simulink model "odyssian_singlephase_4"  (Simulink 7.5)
settings: Solver=ode23t  StartTime=0.0  StopTime=6  RelTol=1e-6
undefined symbols (not defined in the file or in its folder): dfilt, DiscIntNeverNeededParam
libraries: powerlib x72, powerlib_extras x29, simulink x24, dsparch4 x4
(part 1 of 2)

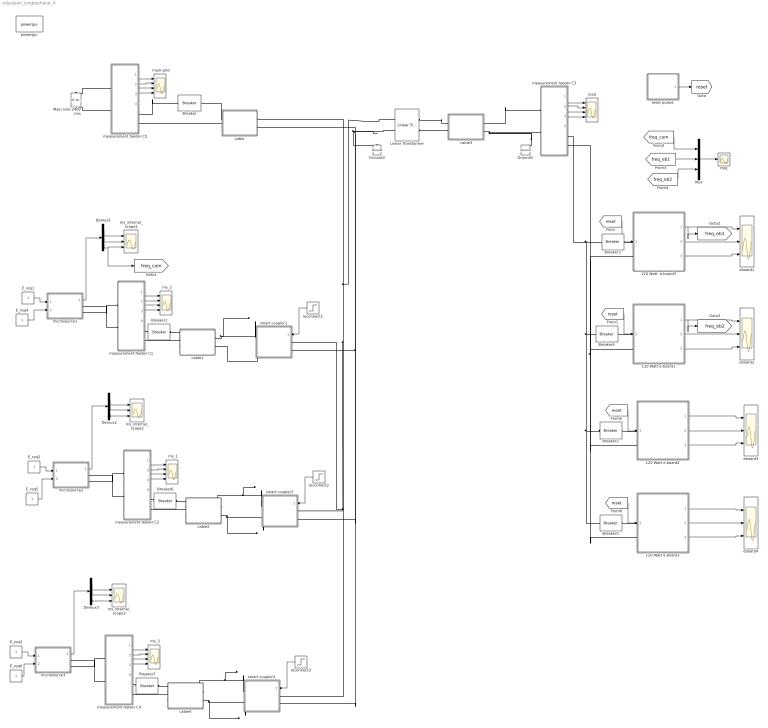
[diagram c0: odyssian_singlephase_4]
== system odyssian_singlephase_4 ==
  " load" : Scope  NumInputPorts=4
  " main-grid" : Scope  NumInputPorts=4
  " ms_1" : Scope  NumInputPorts=4
  " ms_2" : Scope  NumInputPorts=4
  " ms_3" : Scope  NumInputPorts=4
  120 Watt  e-board3 : Subsystem  mask{tf=100, p=1}
      mask prompts: tf "fault_time"; p "load priority"
  120 Watt e-board1 : Subsystem  mask{tf=100, p=1}
      mask prompts: tf "fault_time"; p "load priority"
  120 Watt e-board2 : Subsystem  mask{tf=100, p=1}
      mask prompts: tf "fault_time"; p "load priority"
  120 Watt e-board3 : Subsystem  mask{tf=100, p=2}
      mask prompts: tf "fault_time"; p "load priority"
  Breaker : powerlib/Elements/Breaker  DialogController=POWERSYS.PowerSysDialog  SystemSampleTime=-1  BreakerResistance=0.01  InitialState=1  SnubberResistance=1e6  SnubberCapacitance=inf  SwitchingTimes=[3]  External=off  Measurements=None  MoreParameters=off  NoBreakLoop=off
  Breaker{1..6} (6 alike) : powerlib/Elements/Breaker  DialogController=POWERSYS.PowerSysDialog  SystemSampleTime=-1  BreakerResistance=0.01  InitialState=1  SnubberResistance=1e6  SnubberCapacitance=inf  SwitchingTimes=[100]  External=off  Measurements=None  MoreParameters=off  NoBreakLoop=off
  Breaker7 : powerlib/Elements/Breaker  DialogController=POWERSYS.PowerSysDialog  SystemSampleTime=-1  BreakerResistance=0.01  InitialState=1  SnubberResistance=1e6  SnubberCapacitance=inf  SwitchingTimes=[4]  External=off  Measurements=None  MoreParameters=off  NoBreakLoop=off
  Demux1 : Demux  Outputs=3
  Demux2 : Demux  Outputs=3
  Demux3 : Demux  Outputs=3
  E_req{1..6} (6 alike) : Constant  OutDataType=fixdt(1, 16)  OutScaling=2^0
  Ground1 : powerlib/Elements/Ground  DialogController=POWERSYS.PowerSysDialog  PhysicalDomain=powersysdomain  SubClassName=unknown  LeftPortType=p1  RightPortType=p1  LConnTagsString=a
  Ground3 : powerlib/Elements/Ground  DialogController=POWERSYS.PowerSysDialog  PhysicalDomain=powersysdomain  SubClassName=unknown  LeftPortType=p1  RightPortType=p1  LConnTagsString=a
  Linear Transformer : powerlib/Elements/Linear Transformer  DialogController=POWERSYS.PowerSysDialog  PhysicalDomain=powersysdomain  SubClassName=unknown  LeftPortType=p1  RightPortType=p1  LConnTagsString=a|b  RConnTagsString=A|B  UNITS=SI  NominalPower=[ 45e3 , 60 ]  winding1=[240 0.001 1.e-3]  winding2=[120 .001 1.e-3]  ThreeWindings=off  winding3=[3.15e+05 0.7938 0.084225]  RmLm=[1.0804e+06 2866]  Measurements=All voltages and currents  DataType=on
  Main Grid 240V rms : powerlib/Electrical Sources/AC Voltage Source  DialogController=POWERSYS.PowerSysDialog  SystemSampleTime=-1  Amplitude=240*sqrt(2)  Phase=0  Frequency=60  SampleTime=0  Measurements=None
  Mux : Mux  Inputs=3
  cable : Subsystem
  cable1 : Subsystem
  cable2 : Subsystem
  cable3 : Subsystem
  cable4 : Subsystem
  eboard{1..4} (4 alike) : Scope  NumInputPorts=3
  freq : Scope
  measurement feeder C1 : Subsystem
  measurement feeder C2 : Subsystem
  measurement feeder C3 : Subsystem
  measurement feeder C4 : Subsystem
  measurement feeder C5 : Subsystem
  microsource1 : Subsystem  AncestorBlock=|
      | UWM_blocks/inverter-based
      | DG (simplified)
      | 208V - 15kVA
  microsource2 : Subsystem  AncestorBlock=|
      | UWM_blocks/inverter-based
      | DG (simplified)
      | 208V - 15kVA
  microsource3 : Subsystem  AncestorBlock=|
      | UWM_blocks/inverter-based
      | DG (simplified)
      | 208V - 15kVA
  ms_internal_scope1 : Scope  NumInputPorts=3
  ms_internal_scope2 : Scope  NumInputPorts=3
  ms_internal_scope3 : Scope  NumInputPorts=3
  powergui : powerlib/powergui  Priority=1  SystemSampleTime=-1  SimulationMode=Discrete  SampleTime=50e-5  frequency=60  SPID=off  DisableSnubberDevices=off  DisableRonSwitches=off  DisableVfSwitches=off  SwTol=0  Interpol=off  frequencyindice=0  echomessages=off  HookPort=off  DisplayEquations=off  FunctionMessages=off  EnableUseOfTLC=off  x0status=blocks  RestoreLinks=warning  ResistiveCurrentMeasurement=off  Frange=[0:2:500]  Ylog=off  Xlog=on  ShowGrid=off  save=off  variable=ZData  ZoomFFT=on  StartTime=0.0  cycles=1  DisplayStyle=1  fundamental=60  FreqAxis=off  MaxFrequency=1000  frequencyindicesteady=1  RmsSteady=1  display=off  Ts=0  methode=off
  reconnect1 : Step  Time=.1  SampleTime=0
  reconnect2 : Step  Time=.1  SampleTime=0
  reconnect3 : Step  Time=.1  SampleTime=0
  reset pulses : Subsystem  mask{tpulse=[50 100]}
  smart coupler1 : Subsystem
  smart coupler2 : Subsystem
  smart coupler3 : Subsystem
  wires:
  measurement feeder C3/1(Vm) -> " load"/1
  measurement feeder C3/2(Im) -> " load"/2
  measurement feeder C3/3(PQ) -> " load"/3
  measurement feeder C3/4(RMS (V-I)) -> " load"/4
  120 Watt  e-board3/1(w) -> eboard1/1, [freq_eb1]
  120 Watt  e-board3/2(Irms) -> eboard1/2
  120 Watt  e-board3/3(Vrms) -> eboard1/3
  [reset] -> 120 Watt  e-board3/1(reset)
  120 Watt e-board1/1(w) -> eboard2/1, [freq_eb2]
  120 Watt e-board1/2(Irms) -> eboard2/2
  120 Watt e-board1/3(Vrms) -> eboard2/3
  [reset] -> 120 Watt e-board1/1(reset)
  Mux/1 -> freq/1
  reset pulses/1(Out1) -> [reset]
  [freq_com] -> Mux/1
  [freq_eb1] -> Mux/2
  [freq_eb2] -> Mux/3
  measurement feeder C5/1(Vm) -> " main-grid"/1
  measurement feeder C5/2(Im) -> " main-grid"/2
  measurement feeder C5/3(PQ) -> " main-grid"/3
  measurement feeder C5/4(RMS (V-I)) -> " main-grid"/4
  measurement feeder C1/1(Vm) -> " ms_2"/1
  measurement feeder C1/2(Im) -> " ms_2"/2
  measurement feeder C1/3(PQ) -> " ms_2"/3
  measurement feeder C1/4(RMS (V-I)) -> " ms_2"/4
  E_req1/1 -> microsource1/1(E_req)
  Demux1/2 -> ms_internal_scope1/2
  Demux1/1 -> ms_internal_scope1/1
  Demux1/3 -> ms_internal_scope1/3, [freq_com]
  microsource1/1(m) -> Demux1/1
  reconnect1/1 -> smart coupler1/1(switch)
  ? -> ?
  120 Watt e-board2/1(w) -> eboard3/1
  120 Watt e-board2/2(Irms) -> eboard3/2
  120 Watt e-board2/3(Vrms) -> eboard3/3
  [reset] -> 120 Watt e-board2/1(reset)
  120 Watt e-board3/1(w) -> eboard4/1
  120 Watt e-board3/2(Irms) -> eboard4/2
  120 Watt e-board3/3(Vrms) -> eboard4/3
  [reset] -> 120 Watt e-board3/1(reset)
  measurement feeder C2/1(Vm) -> " ms_1"/1
  measurement feeder C2/2(Im) -> " ms_1"/2
  measurement feeder C2/3(PQ) -> " ms_1"/3
  measurement feeder C2/4(RMS (V-I)) -> " ms_1"/4
  E_req2/1 -> microsource2/1(E_req)
  Demux2/2 -> ms_internal_scope2/2
  Demux2/1 -> ms_internal_scope2/1
  Demux2/3 -> ms_internal_scope2/3
  microsource2/1(m) -> Demux2/1
  reconnect2/1 -> smart coupler2/1(switch)
  measurement feeder C4/1(Vm) -> " ms_3"/1
  measurement feeder C4/2(Im) -> " ms_3"/2
  measurement feeder C4/3(PQ) -> " ms_3"/3
  measurement feeder C4/4(RMS (V-I)) -> " ms_3"/4
  E_req3/1 -> microsource3/1(E_req)
  Demux3/2 -> ms_internal_scope3/2
  Demux3/1 -> ms_internal_scope3/1
  Demux3/3 -> ms_internal_scope3/3
  microsource3/1(m) -> Demux3/1
  reconnect3/1 -> smart coupler3/1(switch)
  E_req4/1 -> microsource1/2(P_req)
  E_req5/1 -> microsource2/2(P_req)
  E_req6/1 -> microsource3/2(P_req)
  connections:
  Breaker2/RConn1 -- Breaker4/RConn1 -- measurement feeder C3/RConn1 -- Breaker3/RConn1 -- Breaker5/RConn1
  measurement feeder C3/RConn2 -- 120 Watt  e-board3/LConn2 -- 120 Watt e-board1/LConn2 -- 120 Watt e-board2/LConn2 -- 120 Watt e-board3/LConn2
  cable3/LConn2 -- Ground1/LConn1 -- measurement feeder C3/LConn2
  120 Watt  e-board3/LConn1 -- Breaker3/LConn1
  120 Watt e-board1/LConn1 -- Breaker4/LConn1
  measurement feeder C5/RConn1 -- Breaker/LConn1
  cable/RConn2 -- measurement feeder C5/RConn2
  cable/RConn1 -- Breaker/RConn1
  smart coupler1/LConn1 -- Linear Transformer/LConn1 -- cable/LConn1 -- smart coupler2/LConn1 -- smart coupler3/LConn1
  Linear Transformer/LConn2 -- Ground3/LConn1 -- cable/LConn2 -- smart coupler1/LConn2 -- smart coupler2/LConn2 -- smart coupler3/LConn2
  cable3/LConn1 -- measurement feeder C3/LConn1
  cable3/RConn2 -- Linear Transformer/RConn2
  cable3/RConn1 -- Linear Transformer/RConn1
  measurement feeder C5/LConn1 -- Main Grid 240V rms/RConn1
  measurement feeder C5/LConn2 -- Main Grid 240V rms/LConn1
  smart coupler1/RConn2 -- cable1/LConn2
  cable1/LConn1 -- smart coupler1/RConn1
  cable1/RConn2 -- measurement feeder C1/RConn2
  measurement feeder C1/LConn1 -- microsource1/RConn1
  cable1/RConn1 -- Breaker1/LConn1
  measurement feeder C1/LConn2 -- microsource1/RConn2
  Breaker1/RConn1 -- measurement feeder C1/RConn1
  120 Watt e-board2/LConn1 -- Breaker2/LConn1
  120 Watt e-board3/LConn1 -- Breaker5/LConn1
  cable2/LConn2 -- smart coupler2/RConn2
  cable2/LConn1 -- smart coupler2/RConn1
  cable2/RConn2 -- measurement feeder C2/RConn2
  measurement feeder C2/LConn1 -- microsource2/RConn1
  cable2/RConn1 -- Breaker6/LConn1
  measurement feeder C2/LConn2 -- microsource2/RConn2
  Breaker6/RConn1 -- measurement feeder C2/RConn1
  cable4/LConn2 -- smart coupler3/RConn2
  cable4/LConn1 -- smart coupler3/RConn1
  cable4/RConn2 -- measurement feeder C4/RConn2
  measurement feeder C4/LConn1 -- microsource3/RConn1
  cable4/RConn1 -- Breaker7/LConn1
  measurement feeder C4/LConn2 -- microsource3/RConn2
  Breaker7/RConn1 -- measurement feeder C4/RConn1

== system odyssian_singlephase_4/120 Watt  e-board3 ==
  reset : Inport
  Breaker : powerlib/Elements/Breaker  DialogController=POWERSYS.PowerSysDialog  SystemSampleTime=-1  BreakerResistance=0.01  InitialState=1  SnubberResistance=1e6  SnubberCapacitance=inf  SwitchingTimes="[ 1/60  5/60 ]"  External=on  Measurements=None  MoreParameters=off  NoBreakLoop=off
  Current Measurement : powerlib/Measurements/Current Measurement  DialogController=POWERSYS.PowerSysDialog  SystemSampleTime=-1  PhasorSimulation=off  OutputType=Complex  PSBequivalent=0
  Ground : powerlib/Elements/Ground  DialogController=POWERSYS.PowerSysDialog  PhysicalDomain=powersysdomain  SubClassName=unknown  LeftPortType=p1  RightPortType=p1  LConnTagsString=a
  Series RLC Load : powerlib/Elements/Series RLC Load  DialogController=POWERSYS.PowerSysDialog  PhysicalDomain=powersysdomain  SubClassName=unknown  LeftPortType=p1  RightPortType=p1  LConnTagsString=a  RConnTagsString=__new0  NominalVoltage=120  NominalFrequency=60  ActivePower=120  InductivePower=0  CapacitivePower=0  Setx0=off  InitialVoltage=0  SetiL0=off  InitialCurrent=0  Measurements=None
  Voltage  Measurement : powerlib/Measurements/Voltage Measurement  DialogController=POWERSYS.PowerSysDialog  SystemSampleTime=-1  PhasorSimulation=off  OutputType=Complex  PSBequivalent=0
  trip : Subsystem  mask{p=p}
      mask prompts: p "priority level"
  A : PMIOPort  Port=1  Side=Left
  C : PMIOPort  Port=2  Side=Left
  w : Outport  OutDataType=fixdt(1, 16)  OutScaling=2^0
  Irms : Outport  Port=2  OutDataType=fixdt(1, 16)  OutScaling=2^0
  Vrms : Outport  Port=3  OutDataType=fixdt(1, 16)  OutScaling=2^0
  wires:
  trip/1(w) -> w/1
  Current Measurement/1 -> trip/3(I)
  Voltage  Measurement/1 -> trip/2(V)
  reset/1 -> trip/1(Reset)
  trip/2(trip) -> Breaker/1
  trip/3(Irms) -> Irms/1
  trip/4(Vrms) -> Vrms/1
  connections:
  A/RConn1 -- Current Measurement/LConn1 -- Voltage  Measurement/LConn1
  Voltage  Measurement/LConn2 -- Ground/LConn1
  Current Measurement/RConn1 -- Breaker/LConn1
  Series RLC Load/LConn1 -- Breaker/RConn1
  Series RLC Load/RConn1 -- C/RConn1

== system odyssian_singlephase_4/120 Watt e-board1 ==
  reset : Inport
  Breaker : powerlib/Elements/Breaker  DialogController=POWERSYS.PowerSysDialog  SystemSampleTime=-1  BreakerResistance=0.01  InitialState=1  SnubberResistance=1e6  SnubberCapacitance=inf  SwitchingTimes="[ 1/60  5/60 ]"  External=on  Measurements=None  MoreParameters=off  NoBreakLoop=off
  Current Measurement : powerlib/Measurements/Current Measurement  DialogController=POWERSYS.PowerSysDialog  SystemSampleTime=-1  PhasorSimulation=off  OutputType=Complex  PSBequivalent=0
  Ground : powerlib/Elements/Ground  DialogController=POWERSYS.PowerSysDialog  PhysicalDomain=powersysdomain  SubClassName=unknown  LeftPortType=p1  RightPortType=p1  LConnTagsString=a
  Series RLC Load : powerlib/Elements/Series RLC Load  DialogController=POWERSYS.PowerSysDialog  PhysicalDomain=powersysdomain  SubClassName=unknown  LeftPortType=p1  RightPortType=p1  LConnTagsString=a  RConnTagsString=__new0  NominalVoltage=120  NominalFrequency=60  ActivePower=120  InductivePower=0  CapacitivePower=0  Setx0=off  InitialVoltage=0  SetiL0=off  InitialCurrent=0  Measurements=None
  Voltage  Measurement : powerlib/Measurements/Voltage Measurement  DialogController=POWERSYS.PowerSysDialog  SystemSampleTime=-1  PhasorSimulation=off  OutputType=Complex  PSBequivalent=0
  trip : Subsystem  mask{p=p}
      mask prompts: p "priority level"
  A : PMIOPort  Port=1  Side=Left
  C : PMIOPort  Port=2  Side=Left
  w : Outport  OutDataType=fixdt(1, 16)  OutScaling=2^0
  Irms : Outport  Port=2  OutDataType=fixdt(1, 16)  OutScaling=2^0
  Vrms : Outport  Port=3  OutDataType=fixdt(1, 16)  OutScaling=2^0
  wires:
  trip/1(w) -> w/1
  Current Measurement/1 -> trip/3(I)
  Voltage  Measurement/1 -> trip/2(V)
  reset/1 -> trip/1(Reset)
  trip/2(trip) -> Breaker/1
  trip/3(Irms) -> Irms/1
  trip/4(Vrms) -> Vrms/1
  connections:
  A/RConn1 -- Current Measurement/LConn1 -- Voltage  Measurement/LConn1
  Voltage  Measurement/LConn2 -- Ground/LConn1
  Current Measurement/RConn1 -- Breaker/LConn1
  Series RLC Load/LConn1 -- Breaker/RConn1
  Series RLC Load/RConn1 -- C/RConn1

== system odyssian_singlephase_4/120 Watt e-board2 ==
  reset : Inport
  Breaker : powerlib/Elements/Breaker  DialogController=POWERSYS.PowerSysDialog  SystemSampleTime=-1  BreakerResistance=0.01  InitialState=1  SnubberResistance=1e6  SnubberCapacitance=inf  SwitchingTimes="[ 1/60  5/60 ]"  External=on  Measurements=None  MoreParameters=off  NoBreakLoop=off
  Current Measurement : powerlib/Measurements/Current Measurement  DialogController=POWERSYS.PowerSysDialog  SystemSampleTime=-1  PhasorSimulation=off  OutputType=Complex  PSBequivalent=0
  Ground : powerlib/Elements/Ground  DialogController=POWERSYS.PowerSysDialog  PhysicalDomain=powersysdomain  SubClassName=unknown  LeftPortType=p1  RightPortType=p1  LConnTagsString=a
  Series RLC Load : powerlib/Elements/Series RLC Load  DialogController=POWERSYS.PowerSysDialog  PhysicalDomain=powersysdomain  SubClassName=unknown  LeftPortType=p1  RightPortType=p1  LConnTagsString=a  RConnTagsString=__new0  NominalVoltage=120  NominalFrequency=60  ActivePower=120  InductivePower=0  CapacitivePower=0  Setx0=off  InitialVoltage=0  SetiL0=off  InitialCurrent=0  Measurements=None
  Voltage  Measurement : powerlib/Measurements/Voltage Measurement  DialogController=POWERSYS.PowerSysDialog  SystemSampleTime=-1  PhasorSimulation=off  OutputType=Complex  PSBequivalent=0
  trip : Subsystem  mask{p=p}
      mask prompts: p "priority level"
  A : PMIOPort  Port=1  Side=Left
  C : PMIOPort  Port=2  Side=Left
  w : Outport  OutDataType=fixdt(1, 16)  OutScaling=2^0
  Irms : Outport  Port=2  OutDataType=fixdt(1, 16)  OutScaling=2^0
  Vrms : Outport  Port=3  OutDataType=fixdt(1, 16)  OutScaling=2^0
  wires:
  trip/1(w) -> w/1
  Current Measurement/1 -> trip/3(I)
  Voltage  Measurement/1 -> trip/2(V)
  reset/1 -> trip/1(Reset)
  trip/2(trip) -> Breaker/1
  trip/3(Irms) -> Irms/1
  trip/4(Vrms) -> Vrms/1
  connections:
  A/RConn1 -- Current Measurement/LConn1 -- Voltage  Measurement/LConn1
  Voltage  Measurement/LConn2 -- Ground/LConn1
  Current Measurement/RConn1 -- Breaker/LConn1
  Series RLC Load/LConn1 -- Breaker/RConn1
  Series RLC Load/RConn1 -- C/RConn1

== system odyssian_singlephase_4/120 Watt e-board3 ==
  reset : Inport
  Breaker : powerlib/Elements/Breaker  DialogController=POWERSYS.PowerSysDialog  SystemSampleTime=-1  BreakerResistance=0.01  InitialState=1  SnubberResistance=1e6  SnubberCapacitance=inf  SwitchingTimes="[ 1/60  5/60 ]"  External=on  Measurements=None  MoreParameters=off  NoBreakLoop=off
  Current Measurement : powerlib/Measurements/Current Measurement  DialogController=POWERSYS.PowerSysDialog  SystemSampleTime=-1  PhasorSimulation=off  OutputType=Complex  PSBequivalent=0
  Ground : powerlib/Elements/Ground  DialogController=POWERSYS.PowerSysDialog  PhysicalDomain=powersysdomain  SubClassName=unknown  LeftPortType=p1  RightPortType=p1  LConnTagsString=a
  Series RLC Load : powerlib/Elements/Series RLC Load  DialogController=POWERSYS.PowerSysDialog  PhysicalDomain=powersysdomain  SubClassName=unknown  LeftPortType=p1  RightPortType=p1  LConnTagsString=a  RConnTagsString=__new0  NominalVoltage=120  NominalFrequency=60  ActivePower=120  InductivePower=0  CapacitivePower=0  Setx0=off  InitialVoltage=0  SetiL0=off  InitialCurrent=0  Measurements=None
  Voltage  Measurement : powerlib/Measurements/Voltage Measurement  DialogController=POWERSYS.PowerSysDialog  SystemSampleTime=-1  PhasorSimulation=off  OutputType=Complex  PSBequivalent=0
  trip : Subsystem  mask{p=p}
      mask prompts: p "priority level"
  A : PMIOPort  Port=1  Side=Left
  C : PMIOPort  Port=2  Side=Left
  w : Outport  OutDataType=fixdt(1, 16)  OutScaling=2^0
  Irms : Outport  Port=2  OutDataType=fixdt(1, 16)  OutScaling=2^0
  Vrms : Outport  Port=3  OutDataType=fixdt(1, 16)  OutScaling=2^0
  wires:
  trip/1(w) -> w/1
  Current Measurement/1 -> trip/3(I)
  Voltage  Measurement/1 -> trip/2(V)
  reset/1 -> trip/1(Reset)
  trip/2(trip) -> Breaker/1
  trip/3(Irms) -> Irms/1
  trip/4(Vrms) -> Vrms/1
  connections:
  A/RConn1 -- Current Measurement/LConn1 -- Voltage  Measurement/LConn1
  Voltage  Measurement/LConn2 -- Ground/LConn1
  Current Measurement/RConn1 -- Breaker/LConn1
  Series RLC Load/LConn1 -- Breaker/RConn1
  Series RLC Load/RConn1 -- C/RConn1

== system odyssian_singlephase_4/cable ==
  Series RLC Branch : powerlib/Elements/Series RLC Branch  DialogController=POWERSYS.PowerSysDialog  PhysicalDomain=powersysdomain  SubClassName=unknown  LeftPortType=p1  RightPortType=p1  LConnTagsString=__new0  RConnTagsString=__new0  BranchType=RL  Resistance=.001  Inductance=1.e-5  SetiL0=off  InitialCurrent=0  Capacitance=1e-6  Setx0=off  InitialVoltage=0  Measurements=None
  A : PMIOPort  Tag=PMCPort  Port=1  Side=Left
  A' : PMIOPort  Tag=PMCPort  Port=2  Side=Right
  B' : PMIOPort  Tag=PMCPort  Port=3  Side=Right
  B : PMIOPort  Tag=PMCPort  Port=4  Side=Left
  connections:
  A/RConn1 -- Series RLC Branch/LConn1
  A'/RConn1 -- Series RLC Branch/RConn1
  B/RConn1 -- B'/RConn1

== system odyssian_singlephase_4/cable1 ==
  Series RLC Branch : powerlib/Elements/Series RLC Branch  DialogController=POWERSYS.PowerSysDialog  PhysicalDomain=powersysdomain  SubClassName=unknown  LeftPortType=p1  RightPortType=p1  LConnTagsString=__new0  RConnTagsString=__new0  BranchType=RL  Resistance=.001  Inductance=1.e-6  SetiL0=off  InitialCurrent=0  Capacitance=1e-6  Setx0=off  InitialVoltage=0  Measurements=None
  A : PMIOPort  Tag=PMCPort  Port=1  Side=Left
  A' : PMIOPort  Tag=PMCPort  Port=2  Side=Right
  B' : PMIOPort  Tag=PMCPort  Port=3  Side=Right
  B : PMIOPort  Tag=PMCPort  Port=4  Side=Left
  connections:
  A/RConn1 -- Series RLC Branch/LConn1
  Series RLC Branch/RConn1 -- A'/RConn1
  B/RConn1 -- B'/RConn1

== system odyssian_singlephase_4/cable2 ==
  Series RLC Branch : powerlib/Elements/Series RLC Branch  DialogController=POWERSYS.PowerSysDialog  PhysicalDomain=powersysdomain  SubClassName=unknown  LeftPortType=p1  RightPortType=p1  LConnTagsString=__new0  RConnTagsString=__new0  BranchType=RL  Resistance=.001  Inductance=1.e-6  SetiL0=off  InitialCurrent=0  Capacitance=1e-6  Setx0=off  InitialVoltage=0  Measurements=None
  A : PMIOPort  Tag=PMCPort  Port=1  Side=Left
  A' : PMIOPort  Tag=PMCPort  Port=2  Side=Right
  B' : PMIOPort  Tag=PMCPort  Port=3  Side=Right
  B : PMIOPort  Tag=PMCPort  Port=4  Side=Left
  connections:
  A/RConn1 -- Series RLC Branch/LConn1
  Series RLC Branch/RConn1 -- A'/RConn1
  B/RConn1 -- B'/RConn1

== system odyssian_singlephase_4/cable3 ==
  Series RLC Branch : powerlib/Elements/Series RLC Branch  DialogController=POWERSYS.PowerSysDialog  PhysicalDomain=powersysdomain  SubClassName=unknown  LeftPortType=p1  RightPortType=p1  LConnTagsString=__new0  RConnTagsString=__new0  BranchType=RL  Resistance=.001  Inductance=1.e-6  SetiL0=off  InitialCurrent=0  Capacitance=1e-6  Setx0=off  InitialVoltage=0  Measurements=None
  A : PMIOPort  Tag=PMCPort  Port=1  Side=Left
  A' : PMIOPort  Tag=PMCPort  Port=2  Side=Right
  B' : PMIOPort  Tag=PMCPort  Port=3  Side=Right
  B : PMIOPort  Tag=PMCPort  Port=4  Side=Left
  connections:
  A/RConn1 -- Series RLC Branch/LConn1
  Series RLC Branch/RConn1 -- A'/RConn1
  B/RConn1 -- B'/RConn1

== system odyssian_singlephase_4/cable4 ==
  Series RLC Branch : powerlib/Elements/Series RLC Branch  DialogController=POWERSYS.PowerSysDialog  PhysicalDomain=powersysdomain  SubClassName=unknown  LeftPortType=p1  RightPortType=p1  LConnTagsString=__new0  RConnTagsString=__new0  BranchType=RL  Resistance=.001  Inductance=1.e-6  SetiL0=off  InitialCurrent=0  Capacitance=1e-6  Setx0=off  InitialVoltage=0  Measurements=None
  A : PMIOPort  Tag=PMCPort  Port=1  Side=Left
  A' : PMIOPort  Tag=PMCPort  Port=2  Side=Right
  B' : PMIOPort  Tag=PMCPort  Port=3  Side=Right
  B : PMIOPort  Tag=PMCPort  Port=4  Side=Left
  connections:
  A/RConn1 -- Series RLC Branch/LConn1
  Series RLC Branch/RConn1 -- A'/RConn1
  B/RConn1 -- B'/RConn1

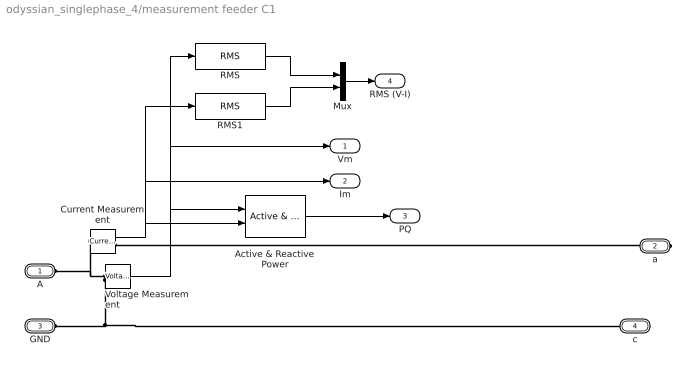
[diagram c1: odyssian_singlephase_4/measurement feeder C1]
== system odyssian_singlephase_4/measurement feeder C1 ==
  Active & Reactive Power : powerlib_extras/Measurements/Active & Reactive Power  DialogController=POWERSYS.PowerSysDialog  SystemSampleTime=-1  f1=60
  Current Measurement : powerlib/Measurements/Current Measurement  DialogController=POWERSYS.PowerSysDialog  SystemSampleTime=-1  PhasorSimulation=off  OutputType=Complex  PSBequivalent=0
  Mux : Mux  Inputs=2
  RMS : powerlib_extras/Measurements/RMS  DialogController=POWERSYS.PowerSysDialog  SystemSampleTime=-1  f1=60
  RMS1 : powerlib_extras/Measurements/RMS  DialogController=POWERSYS.PowerSysDialog  SystemSampleTime=-1  f1=60
  Voltage Measurement : powerlib/Measurements/Voltage Measurement  DialogController=POWERSYS.PowerSysDialog  SystemSampleTime=-1  PhasorSimulation=off  OutputType=Complex  PSBequivalent=0
  A : PMIOPort  Port=1  Side=Left
  a : PMIOPort  Port=2  Side=Right
  GND : PMIOPort  Port=3  Side=Left
  c : PMIOPort  Port=4  Side=Right
  Vm : Outport  OutDataType=fixdt(1, 16)  OutScaling=2^0
  Im : Outport  Port=2  OutDataType=fixdt(1, 16)  OutScaling=2^0
  PQ : Outport  Port=3  OutDataType=fixdt(1, 16)  OutScaling=2^0
  RMS (V-I) : Outport  Port=4  OutDataType=fixdt(1, 16)  OutScaling=2^0
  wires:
  Mux/1 -> RMS (V-I)/1
  Current Measurement/1 -> Im/1, RMS1/1, Active & Reactive Power/2
  Voltage Measurement/1 -> Vm/1, RMS/1, Active & Reactive Power/1
  Active & Reactive Power/1 -> PQ/1
  RMS/1 -> Mux/1
  RMS1/1 -> Mux/2
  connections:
  a/RConn1 -- Current Measurement/RConn1
  Voltage Measurement/LConn1 -- A/RConn1 -- Current Measurement/LConn1
  Voltage Measurement/LConn2 -- GND/RConn1 -- c/RConn1

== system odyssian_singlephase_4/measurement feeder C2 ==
  Active & Reactive Power : powerlib_extras/Measurements/Active & Reactive Power  DialogController=POWERSYS.PowerSysDialog  SystemSampleTime=-1  f1=60
  Current Measurement : powerlib/Measurements/Current Measurement  DialogController=POWERSYS.PowerSysDialog  SystemSampleTime=-1  PhasorSimulation=off  OutputType=Complex  PSBequivalent=0
  Mux : Mux  Inputs=2
  RMS : powerlib_extras/Measurements/RMS  DialogController=POWERSYS.PowerSysDialog  SystemSampleTime=-1  f1=60
  RMS1 : powerlib_extras/Measurements/RMS  DialogController=POWERSYS.PowerSysDialog  SystemSampleTime=-1  f1=60
  Voltage Measurement : powerlib/Measurements/Voltage Measurement  DialogController=POWERSYS.PowerSysDialog  SystemSampleTime=-1  PhasorSimulation=off  OutputType=Complex  PSBequivalent=0
  A : PMIOPort  Port=1  Side=Left
  a : PMIOPort  Port=2  Side=Right
  GND : PMIOPort  Port=3  Side=Left
  c : PMIOPort  Port=4  Side=Right
  Vm : Outport  OutDataType=fixdt(1, 16)  OutScaling=2^0
  Im : Outport  Port=2  OutDataType=fixdt(1, 16)  OutScaling=2^0
  PQ : Outport  Port=3  OutDataType=fixdt(1, 16)  OutScaling=2^0
  RMS (V-I) : Outport  Port=4  OutDataType=fixdt(1, 16)  OutScaling=2^0
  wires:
  Mux/1 -> RMS (V-I)/1
  Current Measurement/1 -> Im/1, RMS1/1, Active & Reactive Power/2
  Voltage Measurement/1 -> Vm/1, RMS/1, Active & Reactive Power/1
  Active & Reactive Power/1 -> PQ/1
  RMS/1 -> Mux/1
  RMS1/1 -> Mux/2
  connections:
  a/RConn1 -- Current Measurement/RConn1
  Voltage Measurement/LConn1 -- A/RConn1 -- Current Measurement/LConn1
  Voltage Measurement/LConn2 -- GND/RConn1 -- c/RConn1

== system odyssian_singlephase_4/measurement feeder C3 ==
  Active & Reactive Power : powerlib_extras/Measurements/Active & Reactive Power  DialogController=POWERSYS.PowerSysDialog  SystemSampleTime=-1  f1=60
  Current Measurement : powerlib/Measurements/Current Measurement  DialogController=POWERSYS.PowerSysDialog  SystemSampleTime=-1  PhasorSimulation=off  OutputType=Complex  PSBequivalent=0
  Mux : Mux  Inputs=2
  RMS : powerlib_extras/Measurements/RMS  DialogController=POWERSYS.PowerSysDialog  SystemSampleTime=-1  f1=60
  RMS1 : powerlib_extras/Measurements/RMS  DialogController=POWERSYS.PowerSysDialog  SystemSampleTime=-1  f1=60
  Voltage Measurement : powerlib/Measurements/Voltage Measurement  DialogController=POWERSYS.PowerSysDialog  SystemSampleTime=-1  PhasorSimulation=off  OutputType=Complex  PSBequivalent=0
  A : PMIOPort  Port=1  Side=Left
  a : PMIOPort  Port=2  Side=Right
  GND : PMIOPort  Port=3  Side=Left
  c : PMIOPort  Port=4  Side=Right
  Vm : Outport  OutDataType=fixdt(1, 16)  OutScaling=2^0
  Im : Outport  Port=2  OutDataType=fixdt(1, 16)  OutScaling=2^0
  PQ : Outport  Port=3  OutDataType=fixdt(1, 16)  OutScaling=2^0
  RMS (V-I) : Outport  Port=4  OutDataType=fixdt(1, 16)  OutScaling=2^0
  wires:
  Mux/1 -> RMS (V-I)/1
  Current Measurement/1 -> Im/1, RMS1/1, Active & Reactive Power/2
  Voltage Measurement/1 -> Vm/1, RMS/1, Active & Reactive Power/1
  Active & Reactive Power/1 -> PQ/1
  RMS/1 -> Mux/1
  RMS1/1 -> Mux/2
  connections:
  a/RConn1 -- Current Measurement/RConn1
  Voltage Measurement/LConn1 -- A/RConn1 -- Current Measurement/LConn1
  Voltage Measurement/LConn2 -- GND/RConn1 -- c/RConn1

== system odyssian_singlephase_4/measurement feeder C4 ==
  Active & Reactive Power : powerlib_extras/Measurements/Active & Reactive Power  DialogController=POWERSYS.PowerSysDialog  SystemSampleTime=-1  f1=60
  Current Measurement : powerlib/Measurements/Current Measurement  DialogController=POWERSYS.PowerSysDialog  SystemSampleTime=-1  PhasorSimulation=off  OutputType=Complex  PSBequivalent=0
  Mux : Mux  Inputs=2
  RMS : powerlib_extras/Measurements/RMS  DialogController=POWERSYS.PowerSysDialog  SystemSampleTime=-1  f1=60
  RMS1 : powerlib_extras/Measurements/RMS  DialogController=POWERSYS.PowerSysDialog  SystemSampleTime=-1  f1=60
  Voltage Measurement : powerlib/Measurements/Voltage Measurement  DialogController=POWERSYS.PowerSysDialog  SystemSampleTime=-1  PhasorSimulation=off  OutputType=Complex  PSBequivalent=0
  A : PMIOPort  Port=1  Side=Left
  a : PMIOPort  Port=2  Side=Right
  GND : PMIOPort  Port=3  Side=Left
  c : PMIOPort  Port=4  Side=Right
  Vm : Outport  OutDataType=fixdt(1, 16)  OutScaling=2^0
  Im : Outport  Port=2  OutDataType=fixdt(1, 16)  OutScaling=2^0
  PQ : Outport  Port=3  OutDataType=fixdt(1, 16)  OutScaling=2^0
  RMS (V-I) : Outport  Port=4  OutDataType=fixdt(1, 16)  OutScaling=2^0
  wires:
  Mux/1 -> RMS (V-I)/1
  Current Measurement/1 -> Im/1, RMS1/1, Active & Reactive Power/2
  Voltage Measurement/1 -> Vm/1, RMS/1, Active & Reactive Power/1
  Active & Reactive Power/1 -> PQ/1
  RMS/1 -> Mux/1
  RMS1/1 -> Mux/2
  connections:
  a/RConn1 -- Current Measurement/RConn1
  Voltage Measurement/LConn1 -- A/RConn1 -- Current Measurement/LConn1
  Voltage Measurement/LConn2 -- GND/RConn1 -- c/RConn1

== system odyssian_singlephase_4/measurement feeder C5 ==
  Active & Reactive Power : powerlib_extras/Measurements/Active & Reactive Power  DialogController=POWERSYS.PowerSysDialog  SystemSampleTime=-1  f1=60
  Current Measurement : powerlib/Measurements/Current Measurement  DialogController=POWERSYS.PowerSysDialog  SystemSampleTime=-1  PhasorSimulation=off  OutputType=Complex  PSBequivalent=0
  Mux : Mux  Inputs=2
  RMS : powerlib_extras/Measurements/RMS  DialogController=POWERSYS.PowerSysDialog  SystemSampleTime=-1  f1=60
  RMS1 : powerlib_extras/Measurements/RMS  DialogController=POWERSYS.PowerSysDialog  SystemSampleTime=-1  f1=60
  Voltage Measurement : powerlib/Measurements/Voltage Measurement  DialogController=POWERSYS.PowerSysDialog  SystemSampleTime=-1  PhasorSimulation=off  OutputType=Complex  PSBequivalent=0
  A : PMIOPort  Port=1  Side=Left
  a : PMIOPort  Port=2  Side=Right
  GND : PMIOPort  Port=3  Side=Left
  c : PMIOPort  Port=4  Side=Right
  Vm : Outport  OutDataType=fixdt(1, 16)  OutScaling=2^0
  Im : Outport  Port=2  OutDataType=fixdt(1, 16)  OutScaling=2^0
  PQ : Outport  Port=3  OutDataType=fixdt(1, 16)  OutScaling=2^0
  RMS (V-I) : Outport  Port=4  OutDataType=fixdt(1, 16)  OutScaling=2^0
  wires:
  Mux/1 -> RMS (V-I)/1
  Current Measurement/1 -> Im/1, RMS1/1, Active & Reactive Power/2
  Voltage Measurement/1 -> Vm/1, RMS/1, Active & Reactive Power/1
  Active & Reactive Power/1 -> PQ/1
  RMS/1 -> Mux/1
  RMS1/1 -> Mux/2
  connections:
  a/RConn1 -- Current Measurement/RConn1
  Voltage Measurement/LConn1 -- A/RConn1 -- Current Measurement/LConn1
  Voltage Measurement/LConn2 -- GND/RConn1 -- c/RConn1

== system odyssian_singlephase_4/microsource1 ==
  E_req : Inport
  P_req : Inport  Port=2
  Current Measurement : powerlib/Measurements/Current Measurement  DialogController=POWERSYS.PowerSysDialog  SystemSampleTime=-1  PhasorSimulation=off  OutputType=Complex  PSBequivalent=0
  Gain : Gain  Gain=1/(2*pi)  ParameterDataType=fixdt(1, 16)  ParameterScaling=2^0  OutDataType=fixdt(1, 16)  OutScaling=2^0
  Mux : Mux  Inputs=3
  Parallel RLC Branch : powerlib/Elements/Parallel RLC Branch  DialogController=POWERSYS.PowerSysDialog  PhysicalDomain=powersysdomain  SubClassName=unknown  LeftPortType=p1  RightPortType=p1  LConnTagsString=a  RConnTagsString=__new0  BranchType=L  Resistance=1  Inductance=1.e-1  SetiL0=off  InitialCurrent=0  Capacitance=1e-6  Setx0=off  InitialVoltage=0  Measurements=None
  Parallel RLC Branch1 : powerlib/Elements/Parallel RLC Branch  DialogController=POWERSYS.PowerSysDialog  PhysicalDomain=powersysdomain  SubClassName=unknown  LeftPortType=p1  RightPortType=p1  LConnTagsString=a  RConnTagsString=__new0  BranchType=L  Resistance=1  Inductance=1.e-1  SetiL0=off  InitialCurrent=0  Capacitance=1e-6  Setx0=off  InitialVoltage=0  Measurements=None
  Parallel RLC Branch2 : powerlib/Elements/Parallel RLC Branch  DialogController=POWERSYS.PowerSysDialog  PhysicalDomain=powersysdomain  SubClassName=unknown  LeftPortType=p1  RightPortType=p1  LConnTagsString=a  RConnTagsString=__new0  BranchType=C  Resistance=1  Inductance=1.e-1  SetiL0=off  InitialCurrent=0  Capacitance=1.e-5  Setx0=off  InitialVoltage=0  Measurements=None
  UWM_controller : Subsystem  mask{Vbase=240*sqrt(2), Sbase=200}
  Voltage Measurement : powerlib/Measurements/Voltage Measurement  DialogController=POWERSYS.PowerSysDialog  SystemSampleTime=-1  PhasorSimulation=off  OutputType=Complex  PSBequivalent=0
  microsource : Subsystem
  a : PMIOPort  Port=1  Side=Right
  GND : PMIOPort  Port=2  Side=Right
  m : Outport  OutDataType=fixdt(1, 16)  OutScaling=2^0
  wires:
  E_req/1 -> UWM_controller/3(E_req)
  P_req/1 -> UWM_controller/4(P_req)
  UWM_controller/1(Vpk) -> microsource/1(Vpk)
  UWM_controller/2(w) -> microsource/2(w), Gain/1
  Mux/1 -> m/1
  Gain/1 -> Mux/3
  Current Measurement/1 -> Mux/2, UWM_controller/2(i_meas)
  Voltage Measurement/1 -> Mux/1, UWM_controller/1(v_meas)
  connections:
  Voltage Measurement/LConn2 -- GND/RConn1 -- Parallel RLC Branch2/RConn1 -- microsource/RConn2
  Parallel RLC Branch1/RConn1 -- Voltage Measurement/LConn1 -- Current Measurement/LConn1
  a/RConn1 -- Current Measurement/RConn1
  Parallel RLC Branch/LConn1 -- microsource/RConn1
  Parallel RLC Branch2/LConn1 -- Parallel RLC Branch1/LConn1 -- Parallel RLC Branch/RConn1

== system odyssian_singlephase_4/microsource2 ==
  E_req : Inport
  P_req : Inport  Port=2
  Current Measurement : powerlib/Measurements/Current Measurement  DialogController=POWERSYS.PowerSysDialog  SystemSampleTime=-1  PhasorSimulation=off  OutputType=Complex  PSBequivalent=0
  Gain : Gain  Gain=1/(2*pi)  ParameterDataType=fixdt(1, 16)  ParameterScaling=2^0  OutDataType=fixdt(1, 16)  OutScaling=2^0
  Mux : Mux  Inputs=3
  Parallel RLC Branch : powerlib/Elements/Parallel RLC Branch  DialogController=POWERSYS.PowerSysDialog  PhysicalDomain=powersysdomain  SubClassName=unknown  LeftPortType=p1  RightPortType=p1  LConnTagsString=a  RConnTagsString=__new0  BranchType=L  Resistance=1  Inductance=1.e-1  SetiL0=off  InitialCurrent=0  Capacitance=1e-6  Setx0=off  InitialVoltage=0  Measurements=None
  Parallel RLC Branch1 : powerlib/Elements/Parallel RLC Branch  DialogController=POWERSYS.PowerSysDialog  PhysicalDomain=powersysdomain  SubClassName=unknown  LeftPortType=p1  RightPortType=p1  LConnTagsString=a  RConnTagsString=__new0  BranchType=L  Resistance=1  Inductance=1.e-1  SetiL0=off  InitialCurrent=0  Capacitance=1e-6  Setx0=off  InitialVoltage=0  Measurements=None
  Parallel RLC Branch2 : powerlib/Elements/Parallel RLC Branch  DialogController=POWERSYS.PowerSysDialog  PhysicalDomain=powersysdomain  SubClassName=unknown  LeftPortType=p1  RightPortType=p1  LConnTagsString=a  RConnTagsString=__new0  BranchType=C  Resistance=1  Inductance=1.e-1  SetiL0=off  InitialCurrent=0  Capacitance=1.e-5  Setx0=off  InitialVoltage=0  Measurements=None
  UWM_controller : Subsystem  mask{Vbase=240*sqrt(2), Sbase=200}
  Voltage Measurement : powerlib/Measurements/Voltage Measurement  DialogController=POWERSYS.PowerSysDialog  SystemSampleTime=-1  PhasorSimulation=off  OutputType=Complex  PSBequivalent=0
  microsource : Subsystem
  a : PMIOPort  Port=1  Side=Right
  GND : PMIOPort  Port=2  Side=Right
  m : Outport  OutDataType=fixdt(1, 16)  OutScaling=2^0
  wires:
  E_req/1 -> UWM_controller/3(E_req)
  P_req/1 -> UWM_controller/4(P_req)
  UWM_controller/1(Vpk) -> microsource/1(Vpk)
  UWM_controller/2(w) -> microsource/2(w), Gain/1
  Mux/1 -> m/1
  Gain/1 -> Mux/3
  Current Measurement/1 -> Mux/2, UWM_controller/2(i_meas)
  Voltage Measurement/1 -> Mux/1, UWM_controller/1(v_meas)
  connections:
  Voltage Measurement/LConn2 -- GND/RConn1 -- Parallel RLC Branch2/RConn1 -- microsource/RConn2
  Parallel RLC Branch1/RConn1 -- Voltage Measurement/LConn1 -- Current Measurement/LConn1
  a/RConn1 -- Current Measurement/RConn1
  Parallel RLC Branch/LConn1 -- microsource/RConn1
  Parallel RLC Branch2/LConn1 -- Parallel RLC Branch1/LConn1 -- Parallel RLC Branch/RConn1

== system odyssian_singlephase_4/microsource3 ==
  E_req : Inport
  P_req : Inport  Port=2
  Current Measurement : powerlib/Measurements/Current Measurement  DialogController=POWERSYS.PowerSysDialog  SystemSampleTime=-1  PhasorSimulation=off  OutputType=Complex  PSBequivalent=0
  Gain : Gain  Gain=1/(2*pi)  ParameterDataType=fixdt(1, 16)  ParameterScaling=2^0  OutDataType=fixdt(1, 16)  OutScaling=2^0
  Mux : Mux  Inputs=3
  Parallel RLC Branch : powerlib/Elements/Parallel RLC Branch  DialogController=POWERSYS.PowerSysDialog  PhysicalDomain=powersysdomain  SubClassName=unknown  LeftPortType=p1  RightPortType=p1  LConnTagsString=a  RConnTagsString=__new0  BranchType=L  Resistance=1  Inductance=1.e-1  SetiL0=off  InitialCurrent=0  Capacitance=1e-6  Setx0=off  InitialVoltage=0  Measurements=None
  Parallel RLC Branch1 : powerlib/Elements/Parallel RLC Branch  DialogController=POWERSYS.PowerSysDialog  PhysicalDomain=powersysdomain  SubClassName=unknown  LeftPortType=p1  RightPortType=p1  LConnTagsString=a  RConnTagsString=__new0  BranchType=L  Resistance=1  Inductance=1.e-1  SetiL0=off  InitialCurrent=0  Capacitance=1e-6  Setx0=off  InitialVoltage=0  Measurements=None
  Parallel RLC Branch2 : powerlib/Elements/Parallel RLC Branch  DialogController=POWERSYS.PowerSysDialog  PhysicalDomain=powersysdomain  SubClassName=unknown  LeftPortType=p1  RightPortType=p1  LConnTagsString=a  RConnTagsString=__new0  BranchType=C  Resistance=1  Inductance=1.e-1  SetiL0=off  InitialCurrent=0  Capacitance=1.e-5  Setx0=off  InitialVoltage=0  Measurements=None
  UWM_controller : Subsystem  mask{Vbase=240*sqrt(2), Sbase=200}
  Voltage Measurement : powerlib/Measurements/Voltage Measurement  DialogController=POWERSYS.PowerSysDialog  SystemSampleTime=-1  PhasorSimulation=off  OutputType=Complex  PSBequivalent=0
  microsource : Subsystem
  a : PMIOPort  Port=1  Side=Right
  GND : PMIOPort  Port=2  Side=Right
  m : Outport  OutDataType=fixdt(1, 16)  OutScaling=2^0
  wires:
  E_req/1 -> UWM_controller/3(E_req)
  P_req/1 -> UWM_controller/4(P_req)
  UWM_controller/1(Vpk) -> microsource/1(Vpk)
  UWM_controller/2(w) -> microsource/2(w), Gain/1
  Mux/1 -> m/1
  Gain/1 -> Mux/3
  Current Measurement/1 -> Mux/2, UWM_controller/2(i_meas)
  Voltage Measurement/1 -> Mux/1, UWM_controller/1(v_meas)
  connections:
  Voltage Measurement/LConn2 -- GND/RConn1 -- Parallel RLC Branch2/RConn1 -- microsource/RConn2
  Parallel RLC Branch1/RConn1 -- Voltage Measurement/LConn1 -- Current Measurement/LConn1
  a/RConn1 -- Current Measurement/RConn1
  Parallel RLC Branch/LConn1 -- microsource/RConn1
  Parallel RLC Branch2/LConn1 -- Parallel RLC Branch1/LConn1 -- Parallel RLC Branch/RConn1

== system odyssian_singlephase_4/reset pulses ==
  Sum : Sum  Inputs=|++  OutDataType=fixdt(1, 16)  OutScaling=2^0
  pulse : Subsystem  mask{tstart=tpulse(1), dt=.1}
  pulse1 : Subsystem  mask{tstart=tpulse(2), dt=.1}
  Out1 : Outport
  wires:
  pulse/1(Out1) -> Sum/1
  pulse1/1(Out1) -> Sum/2
  Sum/1 -> Out1/1

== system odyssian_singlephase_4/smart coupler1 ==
  switch : Inport  OutDataType=fixdt(1, 16)  OutScaling=2^0
  Abs : Abs  OutDataType=fixdt(1, 16)  OutScaling=2^0
  Breaker : powerlib/Elements/Breaker  DialogController=POWERSYS.PowerSysDialog  SystemSampleTime=-1  BreakerResistance=0.01  InitialState=0  SnubberResistance=1e6  SnubberCapacitance=inf  SwitchingTimes="[ 1/60  5/60 ]"  External=on  Measurements=None  MoreParameters=off  NoBreakLoop=off
  Level-2 M-file S-Function : M-S-Function  FunctionName=smart_coupler
  Scope : Scope  NumInputPorts=3
  Transfer Fcn : TransferFcn  Numerator=[100]  Denominator=[1 100]
  Voltage Measurement : powerlib/Measurements/Voltage Measurement  DialogController=POWERSYS.PowerSysDialog  SystemSampleTime=-1  PhasorSimulation=off  OutputType=Complex  PSBequivalent=0
  A : PMIOPort  Port=1  Side=Left
  C : PMIOPort  Port=2  Side=Left
  a : PMIOPort  Port=3  Side=Right
  c : PMIOPort  Port=4  Side=Right
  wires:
  switch/1 -> Level-2 M-file S-Function/2, Scope/2
  Level-2 M-file S-Function/1 -> Scope/1, Breaker/1
  Voltage Measurement/1 -> Abs/1
  Abs/1 -> Transfer Fcn/1
  Transfer Fcn/1 -> Level-2 M-file S-Function/1, Scope/3
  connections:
  Breaker/LConn1 -- A/RConn1 -- Voltage Measurement/LConn1
  Breaker/RConn1 -- Voltage Measurement/LConn2 -- a/RConn1
  c/RConn1 -- C/RConn1

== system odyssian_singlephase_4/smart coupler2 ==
  switch : Inport  OutDataType=fixdt(1, 16)  OutScaling=2^0
  Abs : Abs  OutDataType=fixdt(1, 16)  OutScaling=2^0
  Breaker : powerlib/Elements/Breaker  DialogController=POWERSYS.PowerSysDialog  SystemSampleTime=-1  BreakerResistance=0.01  InitialState=0  SnubberResistance=1e6  SnubberCapacitance=inf  SwitchingTimes="[ 1/60  5/60 ]"  External=on  Measurements=None  MoreParameters=off  NoBreakLoop=off
  Level-2 M-file S-Function : M-S-Function  FunctionName=smart_coupler
  Scope : Scope  NumInputPorts=3
  Transfer Fcn : TransferFcn  Numerator=[100]  Denominator=[1 100]
  Voltage Measurement : powerlib/Measurements/Voltage Measurement  DialogController=POWERSYS.PowerSysDialog  SystemSampleTime=-1  PhasorSimulation=off  OutputType=Complex  PSBequivalent=0
  A : PMIOPort  Port=1  Side=Left
  C : PMIOPort  Port=2  Side=Left
  a : PMIOPort  Port=3  Side=Right
  c : PMIOPort  Port=4  Side=Right
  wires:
  switch/1 -> Level-2 M-file S-Function/2, Scope/2
  Level-2 M-file S-Function/1 -> Scope/1, Breaker/1
  Voltage Measurement/1 -> Abs/1
  Abs/1 -> Transfer Fcn/1
  Transfer Fcn/1 -> Level-2 M-file S-Function/1, Scope/3
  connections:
  Breaker/LConn1 -- A/RConn1 -- Voltage Measurement/LConn1
  Breaker/RConn1 -- Voltage Measurement/LConn2 -- a/RConn1
  c/RConn1 -- C/RConn1

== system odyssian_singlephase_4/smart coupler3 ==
  switch : Inport  OutDataType=fixdt(1, 16)  OutScaling=2^0
  Abs : Abs  OutDataType=fixdt(1, 16)  OutScaling=2^0
  Breaker : powerlib/Elements/Breaker  DialogController=POWERSYS.PowerSysDialog  SystemSampleTime=-1  BreakerResistance=0.01  InitialState=0  SnubberResistance=1e6  SnubberCapacitance=inf  SwitchingTimes="[ 1/60  5/60 ]"  External=on  Measurements=None  MoreParameters=off  NoBreakLoop=off
  Level-2 M-file S-Function : M-S-Function  FunctionName=smart_coupler
  Scope : Scope  NumInputPorts=3
  Transfer Fcn : TransferFcn  Numerator=[100]  Denominator=[1 100]
  Voltage Measurement : powerlib/Measurements/Voltage Measurement  DialogController=POWERSYS.PowerSysDialog  SystemSampleTime=-1  PhasorSimulation=off  OutputType=Complex  PSBequivalent=0
  A : PMIOPort  Port=1  Side=Left
  C : PMIOPort  Port=2  Side=Left
  a : PMIOPort  Port=3  Side=Right
  c : PMIOPort  Port=4  Side=Right
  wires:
  switch/1 -> Level-2 M-file S-Function/2, Scope/2
  Level-2 M-file S-Function/1 -> Scope/1, Breaker/1
  Voltage Measurement/1 -> Abs/1
  Abs/1 -> Transfer Fcn/1
  Transfer Fcn/1 -> Level-2 M-file S-Function/1, Scope/3
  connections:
  Breaker/LConn1 -- A/RConn1 -- Voltage Measurement/LConn1
  Breaker/RConn1 -- Voltage Measurement/LConn2 -- a/RConn1
  c/RConn1 -- C/RConn1

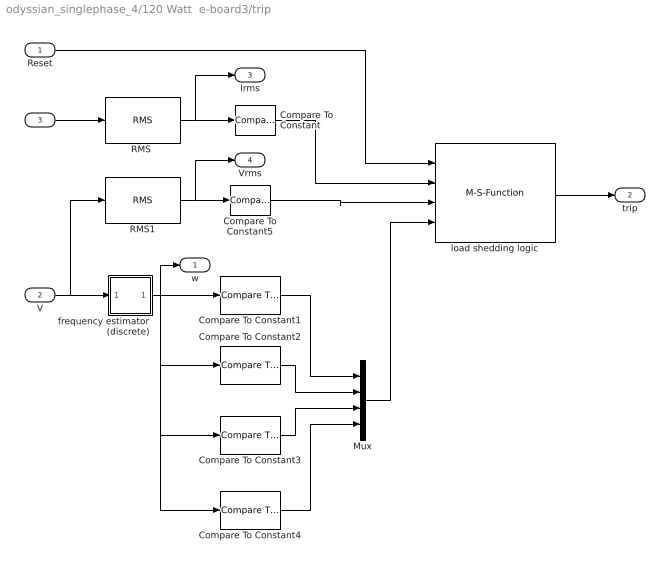
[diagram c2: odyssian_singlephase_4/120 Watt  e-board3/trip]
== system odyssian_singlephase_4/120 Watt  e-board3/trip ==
  Reset : Inport
  V : Inport  Port=2
  I : Inport  Port=3
  Compare To Constant : simulink/Logic and Bit Operations/Compare To Constant  SystemSampleTime=-1  relop=>=  const=100  LogicOutDataTypeMode=boolean
  Compare To Constant1 : simulink/Logic and Bit Operations/Compare To Constant  SystemSampleTime=-1  relop=<=  const=59.8  LogicOutDataTypeMode=boolean
  Compare To Constant2 : simulink/Logic and Bit Operations/Compare To Constant  SystemSampleTime=-1  relop=<=  const=59.5  LogicOutDataTypeMode=boolean
  Compare To Constant3 : simulink/Logic and Bit Operations/Compare To Constant  SystemSampleTime=-1  relop=>=  const=60.1  LogicOutDataTypeMode=boolean
  Compare To Constant4 : simulink/Logic and Bit Operations/Compare To Constant  SystemSampleTime=-1  relop=<=  const=58.6  LogicOutDataTypeMode=boolean
  Compare To Constant5 : simulink/Logic and Bit Operations/Compare To Constant  SystemSampleTime=-1  relop=<=  const=100  LogicOutDataTypeMode=boolean
  Mux : Mux
  "RMS " : powerlib_extras/Measurements/RMS  DialogController=POWERSYS.PowerSysDialog  SystemSampleTime=-1  f1=60
  RMS1 : powerlib_extras/Measurements/RMS  DialogController=POWERSYS.PowerSysDialog  SystemSampleTime=-1  f1=60
  frequency estimator (discrete) : Subsystem  mask{dt=0.010}
      mask prompts: dt "sample time"
  load shedding logic : M-S-Function  FunctionName=load_shedding_logic  Parameters=p
  w : Outport  OutDataType=fixdt(1, 16)  OutScaling=2^0
  trip : Outport  Port=2
  Irms : Outport  Port=3  OutDataType=fixdt(1, 16)  OutScaling=2^0
  Vrms : Outport  Port=4  OutDataType=fixdt(1, 16)  OutScaling=2^0
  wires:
  "RMS "/1 -> Compare To Constant/1, Irms/1
  I/1 -> "RMS "/1
  Reset/1 -> load shedding logic/1
  Compare To Constant/1 -> load shedding logic/2
  load shedding logic/1 -> trip/1
  V/1 -> frequency estimator (discrete)/1(v), RMS1/1
  frequency estimator (discrete)/1(w) -> Compare To Constant1/1, w/1, Compare To Constant2/1, Compare To Constant3/1, Compare To Constant4/1
  Compare To Constant1/1 -> Mux/1
  Compare To Constant2/1 -> Mux/2
  Compare To Constant3/1 -> Mux/3
  Compare To Constant4/1 -> Mux/4
  RMS1/1 -> Compare To Constant5/1, Vrms/1
  Compare To Constant5/1 -> load shedding logic/3
  Mux/1 -> load shedding logic/4

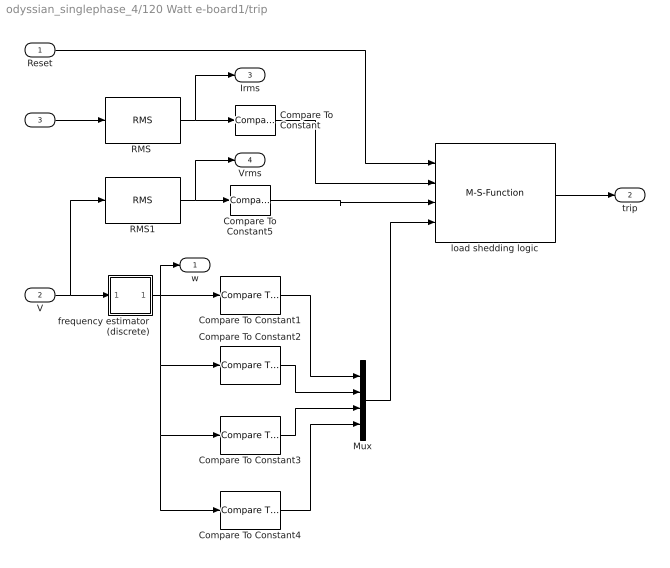
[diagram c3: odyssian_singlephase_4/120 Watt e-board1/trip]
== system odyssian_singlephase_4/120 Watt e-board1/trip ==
  Reset : Inport
  V : Inport  Port=2
  I : Inport  Port=3
  Compare To Constant : simulink/Logic and Bit Operations/Compare To Constant  SystemSampleTime=-1  relop=>=  const=100  LogicOutDataTypeMode=boolean
  Compare To Constant1 : simulink/Logic and Bit Operations/Compare To Constant  SystemSampleTime=-1  relop=<=  const=59.8  LogicOutDataTypeMode=boolean
  Compare To Constant2 : simulink/Logic and Bit Operations/Compare To Constant  SystemSampleTime=-1  relop=<=  const=59.5  LogicOutDataTypeMode=boolean
  Compare To Constant3 : simulink/Logic and Bit Operations/Compare To Constant  SystemSampleTime=-1  relop=>=  const=60.1  LogicOutDataTypeMode=boolean
  Compare To Constant4 : simulink/Logic and Bit Operations/Compare To Constant  SystemSampleTime=-1  relop=<=  const=58.6  LogicOutDataTypeMode=boolean
  Compare To Constant5 : simulink/Logic and Bit Operations/Compare To Constant  SystemSampleTime=-1  relop=<=  const=100  LogicOutDataTypeMode=boolean
  Mux : Mux
  "RMS " : powerlib_extras/Measurements/RMS  DialogController=POWERSYS.PowerSysDialog  SystemSampleTime=-1  f1=60
  RMS1 : powerlib_extras/Measurements/RMS  DialogController=POWERSYS.PowerSysDialog  SystemSampleTime=-1  f1=60
  frequency estimator (discrete) : Subsystem  mask{dt=0.010}
      mask prompts: dt "sample time"
  load shedding logic : M-S-Function  FunctionName=load_shedding_logic  Parameters=p
  w : Outport  OutDataType=fixdt(1, 16)  OutScaling=2^0
  trip : Outport  Port=2
  Irms : Outport  Port=3  OutDataType=fixdt(1, 16)  OutScaling=2^0
  Vrms : Outport  Port=4  OutDataType=fixdt(1, 16)  OutScaling=2^0
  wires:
  "RMS "/1 -> Compare To Constant/1, Irms/1
  I/1 -> "RMS "/1
  Reset/1 -> load shedding logic/1
  Compare To Constant/1 -> load shedding logic/2
  load shedding logic/1 -> trip/1
  V/1 -> frequency estimator (discrete)/1(v), RMS1/1
  frequency estimator (discrete)/1(w) -> Compare To Constant1/1, w/1, Compare To Constant2/1, Compare To Constant3/1, Compare To Constant4/1
  Compare To Constant1/1 -> Mux/1
  Compare To Constant2/1 -> Mux/2
  Compare To Constant3/1 -> Mux/3
  Compare To Constant4/1 -> Mux/4
  RMS1/1 -> Compare To Constant5/1, Vrms/1
  Compare To Constant5/1 -> load shedding logic/3
  Mux/1 -> load shedding logic/4

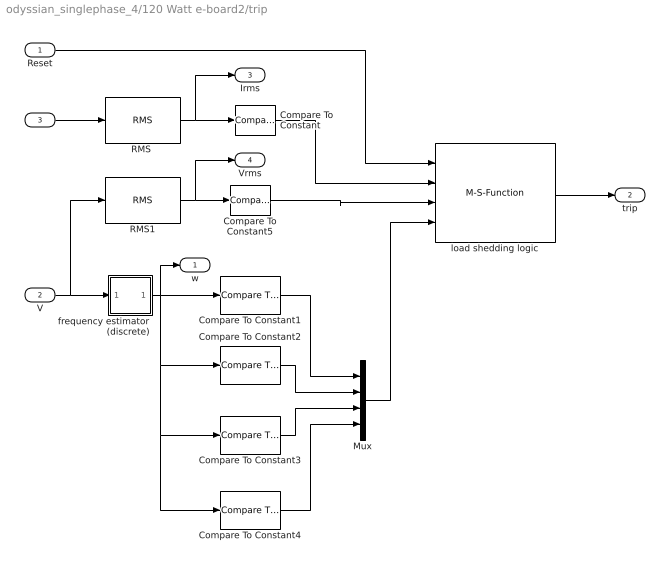
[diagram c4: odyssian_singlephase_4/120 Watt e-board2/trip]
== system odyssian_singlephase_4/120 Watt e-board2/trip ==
  Reset : Inport
  V : Inport  Port=2
  I : Inport  Port=3
  Compare To Constant : simulink/Logic and Bit Operations/Compare To Constant  SystemSampleTime=-1  relop=>=  const=100  LogicOutDataTypeMode=boolean
  Compare To Constant1 : simulink/Logic and Bit Operations/Compare To Constant  SystemSampleTime=-1  relop=<=  const=59.8  LogicOutDataTypeMode=boolean
  Compare To Constant2 : simulink/Logic and Bit Operations/Compare To Constant  SystemSampleTime=-1  relop=<=  const=59.5  LogicOutDataTypeMode=boolean
  Compare To Constant3 : simulink/Logic and Bit Operations/Compare To Constant  SystemSampleTime=-1  relop=>=  const=60.1  LogicOutDataTypeMode=boolean
  Compare To Constant4 : simulink/Logic and Bit Operations/Compare To Constant  SystemSampleTime=-1  relop=<=  const=58.6  LogicOutDataTypeMode=boolean
  Compare To Constant5 : simulink/Logic and Bit Operations/Compare To Constant  SystemSampleTime=-1  relop=<=  const=100  LogicOutDataTypeMode=boolean
  Mux : Mux
  "RMS " : powerlib_extras/Measurements/RMS  DialogController=POWERSYS.PowerSysDialog  SystemSampleTime=-1  f1=60
  RMS1 : powerlib_extras/Measurements/RMS  DialogController=POWERSYS.PowerSysDialog  SystemSampleTime=-1  f1=60
  frequency estimator (discrete) : Subsystem  mask{dt=0.010}
      mask prompts: dt "sample time"
  load shedding logic : M-S-Function  FunctionName=load_shedding_logic  Parameters=p
  w : Outport  OutDataType=fixdt(1, 16)  OutScaling=2^0
  trip : Outport  Port=2
  Irms : Outport  Port=3  OutDataType=fixdt(1, 16)  OutScaling=2^0
  Vrms : Outport  Port=4  OutDataType=fixdt(1, 16)  OutScaling=2^0
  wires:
  "RMS "/1 -> Compare To Constant/1, Irms/1
  I/1 -> "RMS "/1
  Reset/1 -> load shedding logic/1
  Compare To Constant/1 -> load shedding logic/2
  load shedding logic/1 -> trip/1
  V/1 -> frequency estimator (discrete)/1(v), RMS1/1
  frequency estimator (discrete)/1(w) -> Compare To Constant1/1, w/1, Compare To Constant2/1, Compare To Constant3/1, Compare To Constant4/1
  Compare To Constant1/1 -> Mux/1
  Compare To Constant2/1 -> Mux/2
  Compare To Constant3/1 -> Mux/3
  Compare To Constant4/1 -> Mux/4
  RMS1/1 -> Compare To Constant5/1, Vrms/1
  Compare To Constant5/1 -> load shedding logic/3
  Mux/1 -> load shedding logic/4
